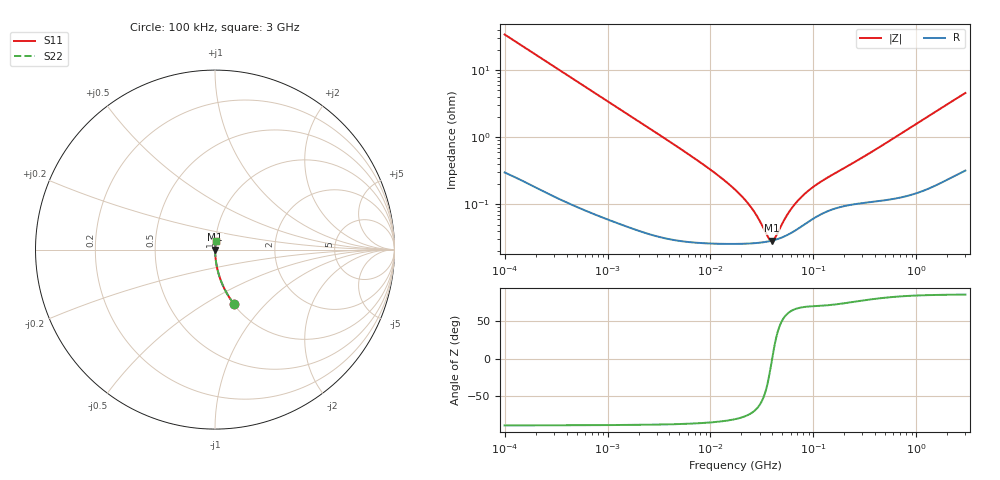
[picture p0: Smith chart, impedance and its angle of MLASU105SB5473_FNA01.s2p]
! MLASU105SB5473_FNA01  S-PARAMETER MODEL  ( Standard Model )
! Model Generated by TAIYO YUDEN Corporation (http://www.ty-top.com)
! Version 1.0
! TAIYO YUDEN Control No. 220601
! Copyright(c) 2014 TAIYO YUDEN CO.,LTD. All Rights Reserved.
! Product Description (link to TY-COMPAS)
! https://ds.yuden.co.jp/TYCOMPAS/or/detail?pn=MLASU105SB5473KFNA01&u=M
! Products Name : Multilayer Ceramic Capacitors
! Characteristics :
!  Capacitance : 0.047 [uF] , Rated Voltage : 50 [V] , TCC : X5R
!  Case Size : 1.0 x 0.5 / 0.039 x 0.02 [mm/inch] , Thickness : 0.5 / 0.02 [mm/inch]
!  (Conditions: Temperature = 25 [degC] , DC Bias Voltage = 0 [V])
! External Node Assignments :
!  1  o---| |---o  2
! GND o---------o GND
! Frequency Range : 100kHz  -  3GHz  [ 401 STEP ]
# MHZ S RI R 50
! Freq[MHz].  S11 Real  S11 Imag  S21 Real  S21 Imag  S12 Real  S12 Imag  S22 Real  S22 Imag
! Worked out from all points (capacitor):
!   401 points, 100 kHz to 3 GHz, reference 50 ohm
!   read as one part in series: C = 46.6 nF near 105.3 kHz
!   lowest |Z| = 28.8 mohm at 39.51 MHz (marker M1)
!   series resonance near 39.78 MHz, so ESL is about 340 pH
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0.1  0.1064 -0.304  0.8936 0.304  0.8936 0.304  0.1064 -0.304
0.147195  0.0532 -0.2195  0.9468 0.2195  0.9468 0.2195  0.0532 -0.2195
0.228123  0.0236 -0.1466  0.9764 0.1466  0.9764 0.1466  0.0236 -0.1466
0.562235  0.00459 -0.061  0.9954 0.061  0.9954 0.061  0.00459 -0.061
1.18716  0.00139 -0.0291  0.9986 0.0291  0.9986 0.0291  0.00139 -0.0291
3.161081  0.000448 -0.011  0.9996 0.011  0.9996 0.011  0.000448 -0.011
9.574722  0.000274 -0.00345  0.9997 0.00345  0.9997 0.00345  0.000274 -0.00345
13.38544  0.000263 -0.00232  0.9997 0.00232  0.9997 0.00232  0.000263 -0.00232
17.7727  0.00026 -0.00158  0.9997 0.00158  0.9997 0.00158  0.00026 -0.00158
21.28644  0.000261 -0.00118  0.9997 0.00118  0.9997 0.00118  0.000261 -0.00118
24.84619  0.000263 -0.000865  0.9997 0.000865  0.9997 0.000865  0.000263 -0.000865
29.00125  0.000267 -0.00057  0.9997 0.00057  0.9997 0.00057  0.000267 -0.00057
36.57227  0.000281 -0.000149  0.9997 0.000149  0.9997 0.000149  0.000281 -0.000149
39.51212  0.000288 -1.18e-05  0.9997 1.18e-05  0.9997 1.18e-05  0.000288 -1.18e-05
42.68829  0.000297 0.000126  0.9997 -0.000126  0.9997 -0.000126  0.000297 0.000126
53.83243  0.000341 0.000543  0.9997 -0.000543  0.9997 -0.000543  0.000341 0.000543
62.83488  0.000387 0.000829  0.9996 -0.000829  0.9996 -0.000829  0.000387 0.000829
77.22239  0.000474 0.00122  0.9995 -0.00122  0.9995 -0.00122  0.000474 0.00122
97.38194  0.000601 0.00167  0.9994 -0.00167  0.9994 -0.00167  0.000601 0.00167
132.6759  0.000778 0.00231  0.9992 -0.00231  0.9992 -0.00231  0.000778 0.00231
547.5153  0.00126 0.00873  0.9987 -0.00873  0.9987 -0.00873  0.00126 0.00873
3000  0.00525 0.0453  0.9947 -0.0453  0.9947 -0.0453  0.00525 0.0453
